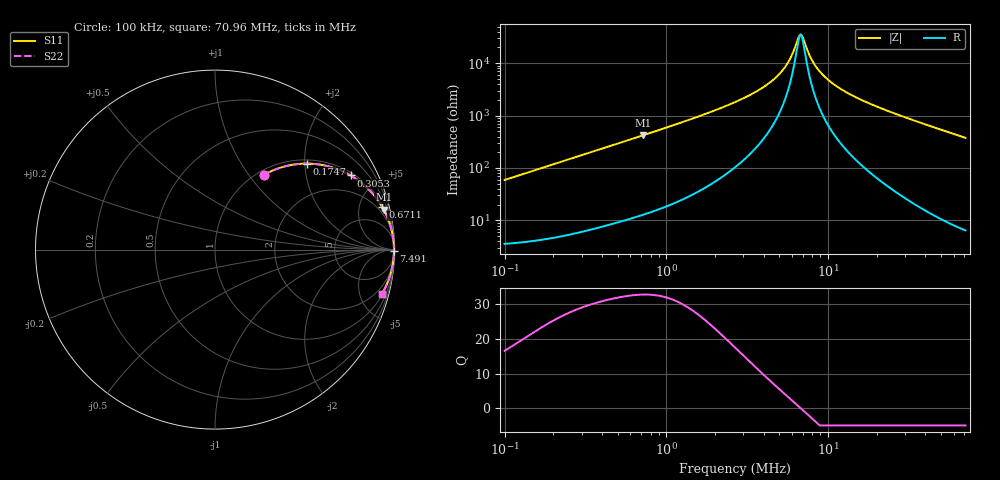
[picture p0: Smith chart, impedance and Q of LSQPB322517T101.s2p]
! LSQPB322517T101  S-PARAMETER MODEL  ( General Type )
! Model Generated by TAIYO YUDEN Corporation (http://www.ty-top.com)
! Version 2.0
! TAIYO YUDEN Control No. 100810NC14SB-FKC
! Copyright(c) 2008 TAIYO YUDEN CO.,LTD. All Rights Reserved.
! Product Description (link to TY-COMPAS)
! https://ds.yuden.co.jp/TYCOMPAS/or/detail?pn=LSQPB322517T101K&u=M
! Products Name : Inductors
! Characteristics :
!  Inductance : 100 uH , SRF(min) : 5.0 MHz , DC Resistance(max) : 3 Ohm
!  Rated Current : Saturation :270 mA , Temp Rise : 250 mA (40 degC)
!  Case Size : 3.2 x 2.5 / 0.126 x 0.098 [mm/inch] , Thickness : 1.7 / 0.068 [mm/inch]
!  (Conditions: Temperature = 25 degC , DC Bias Current/Voltage = 0A / 0V)
! External Node Assignments :
!  1  o---GGG---o  2
! GND o---------o GND
! Frequency Range : 0.1MHz  -  70.9631MHz  [ 402 STEP ]
# MHz S RI R 50
! Freq[MHz].  S11 Real  S11 Imag  S21 Real  S21 Imag  S12 Real  S12 Imag  S22 Real  S22 Imag
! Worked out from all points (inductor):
!   401 points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, 100 kHz to 70.96 MHz, reference 50 ohm
!   read as one part in series: L = 93.9 uH near 103.3 kHz
!   highest Q = 32.9 at 716.7 kHz (marker M1), where L = 93.3 uH
!   self-resonance near 6.678 MHz
!   S11 on the Smith chart (normalised r, x): 100 kHz: 1.07, +1.18; 174.7 kHz: 1.09, +2.06; 305.3 kHz: 1.12, +3.58; 671.1 kHz: 1.24, +7.86; 7.491 MHz: open; 70.96 MHz: 1.13, -7.54
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0.1  0.2715 0.4156  0.7285 -0.4156  0.7285 -0.4156  0.2715 0.4156
0.174718  0.5141 0.4792  0.4859 -0.4792  0.4859 -0.4792  0.5141 0.4792
0.300295  0.7492 0.4166  0.2508 -0.4166  0.2508 -0.4166  0.7492 0.4166
0.305264  0.7551 0.4133  0.2449 -0.4133  0.2449 -0.4133  0.7551 0.4133
0.445256  0.864 0.3272  0.136 -0.3272  0.136 -0.3272  0.864 0.3272
0.671119  0.9329 0.2353  0.0671 -0.2353  0.0671 -0.2353  0.9329 0.2353
0.716654  0.9404 0.2221  0.0596 -0.2221  0.0596 -0.2221  0.9404 0.2221
0.90177  0.9606 0.1798  0.0394 -0.1798  0.0394 -0.1798  0.9606 0.1798
2.70797  0.994 0.0534  0.00599 -0.0534  0.00599 -0.0534  0.994 0.0534
3.822285  0.9961 0.0308  0.00389 -0.0308  0.00389 -0.0308  0.9961 0.0308
4.889189  0.9968 0.017  0.00315 -0.017  0.00315 -0.017  0.9968 0.017
5.761196  0.9971 0.00838  0.00291 -0.00838  0.00291 -0.00838  0.9971 0.00838
6.678222  0.9972 0.000825  0.00282 -0.000825  0.00282 -0.000825  0.9972 0.000825
6.788728  0.9972 -1.01e-05  0.00282 1.01e-05  0.00282 1.01e-05  0.9972 -1.01e-05
7.015257  0.9972 -0.00168  0.00282 0.00168  0.00282 0.00168  0.9972 -0.00168
7.491244  0.9972 -0.00503  0.00283 0.00503  0.00283 0.00503  0.9972 -0.00503
7.999526  0.9971 -0.0084  0.00288 0.0084  0.00288 0.0084  0.9971 -0.0084
9.272834  0.9969 -0.0161  0.00306 0.0161  0.00306 0.0161  0.9969 -0.0161
11.47813  0.9964 -0.028  0.00359 0.028  0.00359 0.028  0.9964 -0.028
15.67816  0.9949 -0.0476  0.00512 0.0476  0.00512 0.0476  0.9949 -0.0476
24.02217  0.9902 -0.0823  0.00978 0.0823  0.00978 0.0823  0.9902 -0.0823
70.9631  0.9307 -0.2455  0.0693 0.2455  0.0693 0.2455  0.9307 -0.2455
